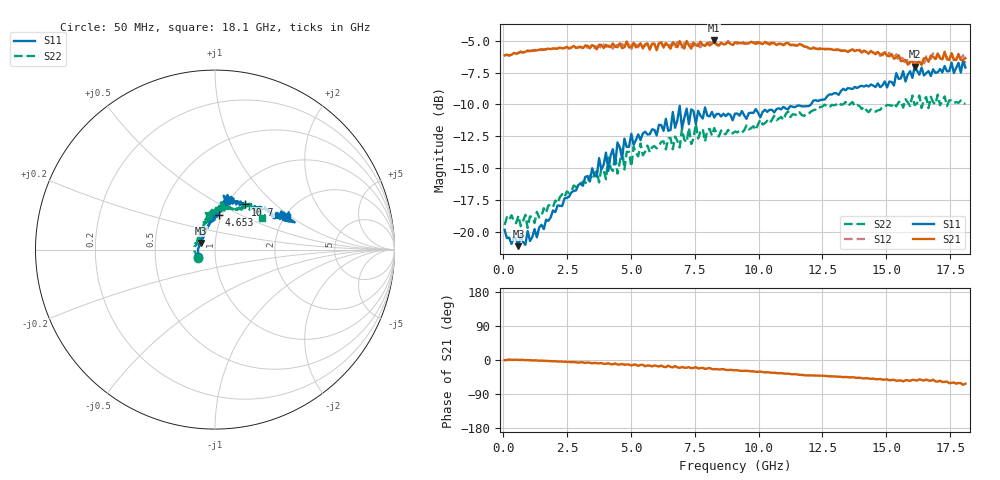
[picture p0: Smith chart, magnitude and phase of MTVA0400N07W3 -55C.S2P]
! Network Analyzer HP8720D.06.14 Serial No. US36140669
!  8 Jul 2005  07:21:00
! Frequency  S11  S21  S12  S22
# HZ  S  DB R 50
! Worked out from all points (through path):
!   201 points, 50 MHz to 18.1 GHz, reference 50 ohm
!   highest |S21| = -4.98 dB at 8.263 GHz (marker M1); lowest = -7.0 dB at 16.11 GHz (marker M2)
!   group delay of S21, straight-line fit = 10.1 ps
!   lowest |S11| = -21.1 dB at 591.5 MHz (marker M3), VSWR 1.19, Z = 42.5 + j3.18 ohm
!   |S11| at or under -10 dB: start of sweep to 12.06 GHz
!   |S22| runs from -19.7 to -9.2 dB; largest |S21 - S12| = 0.036
!   S11 on the Smith chart (normalised r, x): 50 MHz: 0.83, -0.07; 4.653 GHz: 0.97, +0.39; 10.7 GHz: 1.21, +0.67; 18.1 GHz: 2.07, +0.92
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5e7  -19.85 -157.2  -6.16 -0.5  -6.17 -0.3  -19.47 -152.8
5.915e8  -21.13 155.0  -5.97 0.1  -5.93 0.1  -18.75 162.5
9.525e8  -19.95 142.4  -5.77 -0.3  -5.85 -0.0  -19.69 150.5
3.1185e9  -16.39 100.0  -5.59 -6.4  -5.60 -7.0  -16.05 114.1
4.021e9  -13.79 92.0  -5.33 -10.2  -5.49 -8.7  -15.88 104.5
4.382e9  -14.71 88.2  -5.47 -9.3  -5.38 -11.6  -13.93 102.6
4.47225e9  -12.99 82.7  -5.51 -11.9  -5.35 -9.7  -15.43 106.5
4.65275e9  -14.27 82.9  -5.59 -10.4  -5.25 -12.0  -13.52 104.2
4.743e9  -12.69 84.8  -5.50 -12.7  -5.49 -11.0  -15.11 100.4
5.104e9  -13.18 86.5  -5.17 -12.2  -5.26 -13.8  -13.32 94.5
6.09675e9  -11.60 77.9  -5.22 -17.2  -5.14 -16.6  -13.26 89.7
6.7285e9  -11.84 81.8  -5.28 -16.2  -5.63 -17.8  -12.52 82.0
6.909e9  -10.11 77.2  -5.03 -20.8  -5.26 -18.3  -13.38 81.2
6.99925e9  -11.88 77.5  -5.42 -18.1  -5.55 -21.0  -11.92 81.0
7.17975e9  -10.33 80.9  -5.02 -20.3  -5.45 -18.9  -12.98 76.2
8.26275e9  -11.03 73.2  -4.98 -24.4  -5.22 -25.3  -11.86 71.1
9.075e9  -10.72 68.2  -5.16 -26.8  -5.13 -26.9  -12.13 68.7
1.06995e10  -10.37 56.1  -5.34 -34.5  -5.25 -34.3  -11.24 57.4
1.21435e10  -9.71 47.5  -5.57 -40.8  -5.51 -40.7  -10.46 56.5
1.512175e10  -8.20 26.9  -6.23 -53.5  -5.93 -53.0  -10.06 46.7
1.61145e10  -7.01 25.4  -7.03 -52.9  -6.52 -52.8  -10.06 44.6
1.81e10  -7.11 24.1  -6.37 -62.5  -6.76 -62.4  -9.95 34.1
